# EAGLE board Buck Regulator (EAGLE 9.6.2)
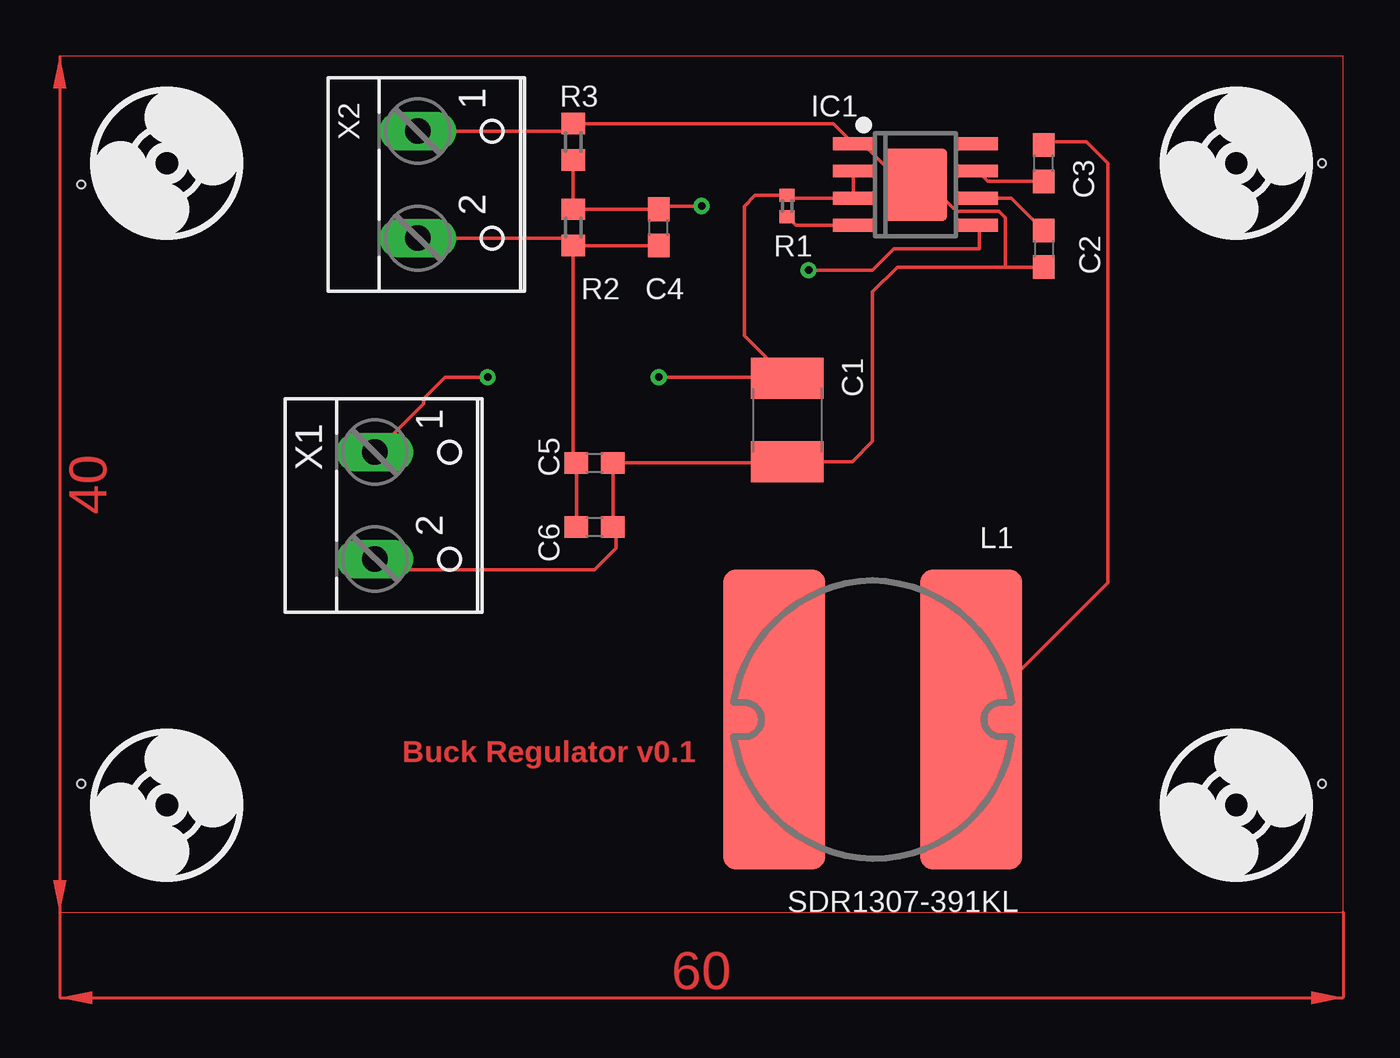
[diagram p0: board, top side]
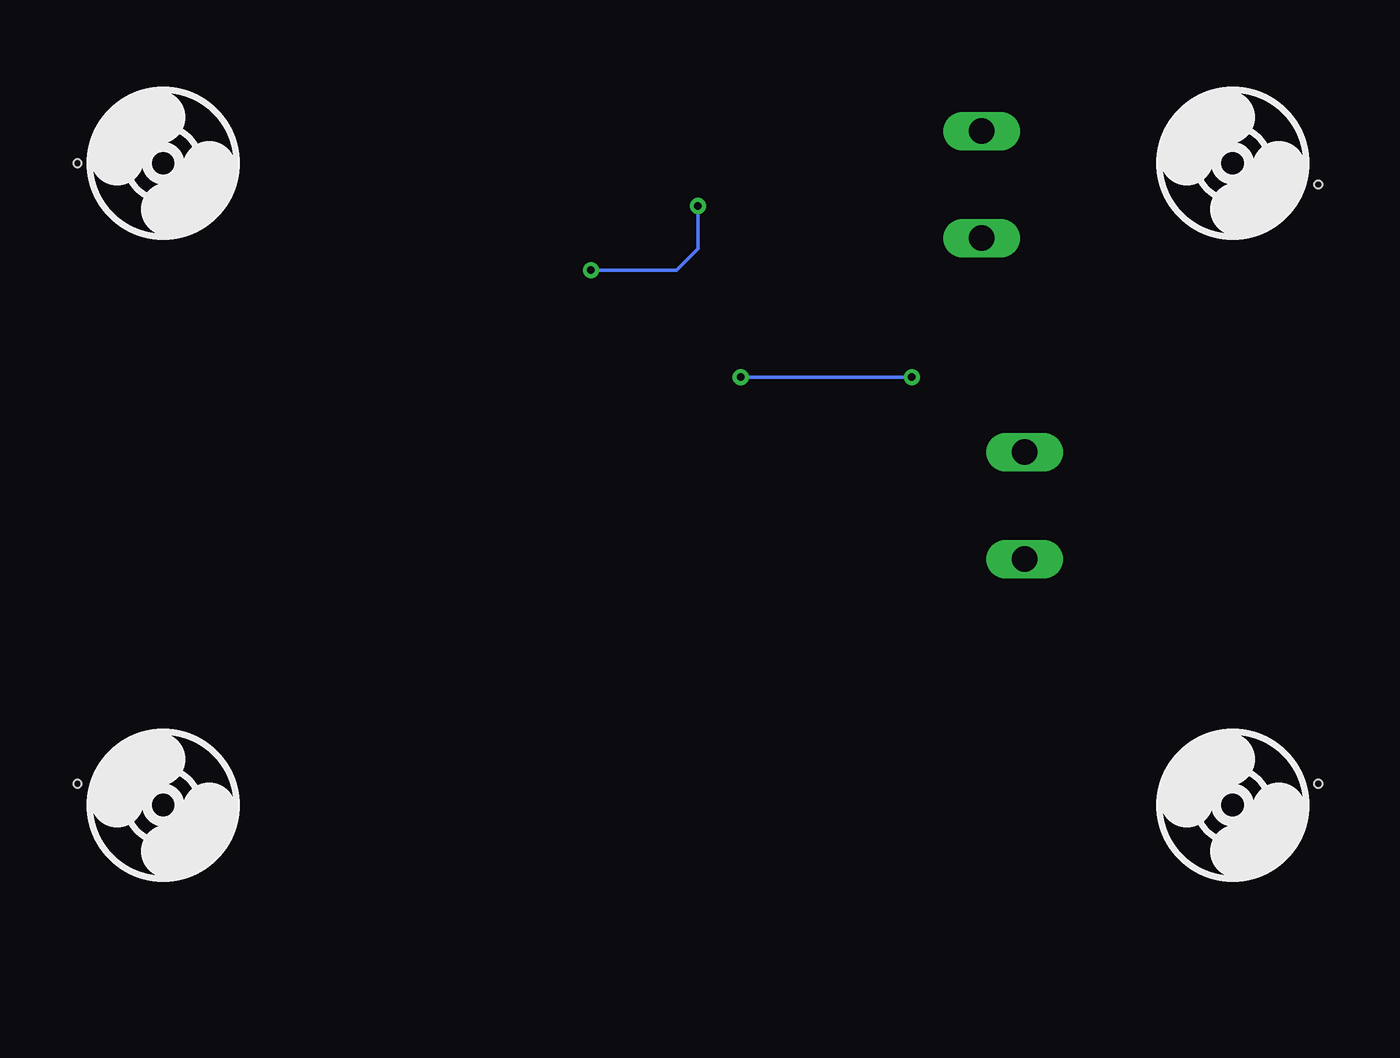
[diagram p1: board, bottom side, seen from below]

No outline drawn. Coordinates in mm, seen from the top.
Copper layers (1*16): Top 0.035mm / dielectric 1.5mm / Bottom 0.035mm
Design rules "default": minimum track width 6mil, minimum drill 0.35mm, track to track 6mil, track to pad 6mil, pad to pad 6mil, via to via 6mil, smd to smd 6mil, copper to edge 40mil, drill to drill 6mil, minimum pad ring 10mil, minimum via ring 8mil, stop-mask expansion 4mil, vias tented up to drill 0mil, thermal gap 10mil
Holes 0.35 mm at 1,34 1,6 59,6 59,35

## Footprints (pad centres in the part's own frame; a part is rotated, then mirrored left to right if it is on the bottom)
C1812 = smd 1.9 x 3.4: 1 -1.95,0; 2 1.95,0
C0603 = smd 1.1 x 1: 1 -0.85,0; 2 0.85,0
3,2 = hole 3.2: 0,0
SO-08-EP = smd 0.6 x 1.9: 1 -1.905,-2.9; 2 -0.635,-2.9; 3 0.635,-2.9; 4 1.905,-2.9; 5 1.905,2.9; 6 0.635,2.9; 7 -0.635,2.9; 8 -1.905,2.9 | smd 3.4 x 2.95: 9 0,0
SDR1307-391KL = smd 14 x 4.75: 1 0,4.6; 2 0,-4.6
R0402 = smd 0.6 x 0.7: 1 -0.5,0; 2 0.5,0
R0603 = smd 1 x 1.1: 1 -0.85,0; 2 0.85,0
W237-102 = drill 1.194 long: 1 -2.5,-1.27; 2 2.5,-1.27

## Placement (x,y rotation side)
C1  2.2uF/150V  [C1812]  34,23 270 top
C2  1uF  [C0603]  46,31 270 top
C3  10nF  [C0603]  46,35 90 top
C4  4.7nF  [C0603]  28,32 90 top
C5  4.7uF  [C0603]  25,21 0 top
C6  4.7uF  [C0603]  25,18 0 top
H1  MOUNT-HOLE3.2  [3,2]  5,5 0 top
H2  MOUNT-HOLE3.2  [3,2]  55,5 180 top
H3  MOUNT-HOLE3.2  [3,2]  55,35 0 top
H4  MOUNT-HOLE3.2  [3,2]  5,35 0 top
IC1  LM5017  [SO-08-EP]  40,34 270 top
L1  SDR1307-391KL  [SDR1307-391KL]  38,9 270 top
R1  499k  [R0402]  34,33 270 top
R2  [R0603]  24,32 270 top
R3  [R0603]  24,36 270 top
X1  [W237-102]  16,19 270 top
X2  [W237-102]  18,34 270 top

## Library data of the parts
C1-C6 = rcl; SPICEPREFIX: C
H1-H4 = _nanolabs_layout
IC1 = _nanolabs_ic
L1 = _nanolabs_rcl
R1-R3 = rcl; SPICEPREFIX: R
X1 X2 = con-wago-500; MPN: 237-102; OC_FARNELL: unknown; OC_NEWARK: 70K9898

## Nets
+12V: C4.1 C5.1 C6.1 R2.2 X2.2
FB: C4.2 IC1.5 R2.1 R3.2
GND: C1.2 C2.2 C5.2 C6.2 IC1.1 IC1.9 R3.1 X1.2 X2.1
N$23: C2.1 IC1.6
N$28: C3.1 IC1.7
N$29: C3.2 L1.1
N$31: IC1.4 R1.2
VIN_HV: C1.1 IC1.2 IC1.3 R1.1 X1.1

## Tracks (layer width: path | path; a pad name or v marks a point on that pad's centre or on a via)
+12V
  Top 0.152: X2.2 23.65,31.5 R2.2 | R2.2 C4.1 | R2.2 24,21.15 C5.1 C6.1
FB  (via drill 0.35)
  Top 0.152: R3.2 R2.1 C4.2 28.15,33 v30,33 | v35,30 38,30 39,31 43,31 43,32 IC1.5
  Bottom 0.152: v35,30 31,30 30,31 v30,33
GND
  Top 0.152: X2.1 23.65,36.5 R3.1 36.16,36.85 IC1.1 37.19,35.81 37.64,35.81 39.32,34.14 39.93,34.14 IC1.9 40.08,33.98 40.69,33.98 41.91,32.77 43.89,32.77 44.2,32.46 44.2,30.15 | 44.2,30.15 39.15,30.15 38,29 38,22 37.05,21.05 C1.2 33.95,21 C5.2 C6.2 26,17.85 26,17 25,16 15.23,16 X1.2 | 44.2,30.15 C2.2
N$23
  Top 0.152: C2.1 44.48,33.37 IC1.6
N$28
  Top 0.152: C3.1 43.38,34.15 IC1.7
N$29
  Top 0.152: C3.2 45.95,35.91 46.04,36 48,36 49,35 49,15.4 L1.1
N$31
  Top 0.152: R1.2 34.41,32.09 IC1.4
S$2
  Top 0: 0,40 0,0
S$3
  Top 0: 60,40 0,40
S$4
  Top 0: 0,0 60,0
S$5
  Top 0: 60,0 60,40
VIN_HV  (via drill 0.35)
  Top 0.152: 33.95,25 32,26.95 32,33 32.5,33.5 R1.1 34.13,33.37 IC1.3 IC1.2 | X1.1 17,23.77 17,24 18,25 v20,25 | v28,25 33.95,25 | 33.95,25 C1.1
  Bottom 0.152: v20,25 v28,25
(copper drawn outside any net)
  shapes: Top area x2

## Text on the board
Top: Buck Regulator v0.1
